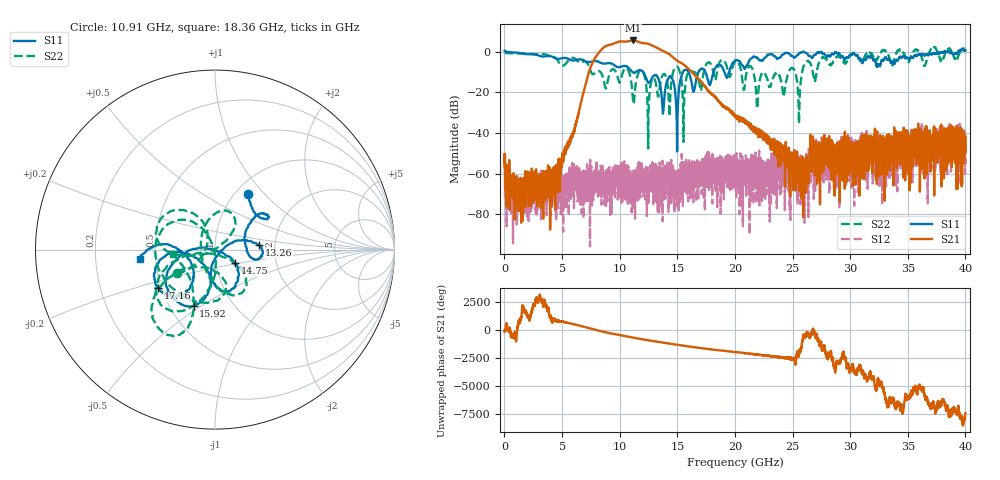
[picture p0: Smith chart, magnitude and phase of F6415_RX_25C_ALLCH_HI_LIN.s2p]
!Keysight Technologies,N5245B,MY52451815,A.15.70.20
!Date: Wednesday, April 17, 2024 14:39:09
!Correction: S33(C  2-Port  )
!S43(C  2-Port  )
!S34(C  2-Port  )
!S44(C  2-Port  )
!S2P File: Measurements: S33, S43, S34, S44:
# Hz S  RI  R 50
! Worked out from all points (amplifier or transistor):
!   4000 points, 10 MHz to 40 GHz, reference 50 ohm
!   highest |S21| = 5.5 dB at 11.15 GHz (marker M1)
!   |S21| within 3 dB of that: 8.712 GHz to 13.02 GHz (4.309 GHz wide, 39.7 % of centre)
!   unconditionally stable (mu >= 1): 139.6 MHz to 25.88 GHz; 25.98 GHz to 32.69 GHz; 35.95 GHz to 36.91 GHz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
!   at 6.67 GHz: K = 4323.53, MAG = -20.5 dB, |S12| = -62.0 dB
!   at 20.01 GHz: K = 8376.42, MAG = -27.7 dB, |S12| = -60.4 dB
!   at 40 GHz: K = 3290.20, MSG = 3.1 dB, |S12| = -55.2 dB
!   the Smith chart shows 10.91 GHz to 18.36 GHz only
!   S11 on the Smith chart (normalised r, x): 10.91 GHz: 1.14, +0.82; 13.26 GHz: 1.64, +0.08; 14.75 GHz: 1.24, -0.19; 15.92 GHz: 0.66, -0.46; 17.16 GHz: 0.48, -0.24; 18.36 GHz: 0.41, -0.05
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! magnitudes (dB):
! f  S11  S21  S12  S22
! 10 MHz  0.5  -54.2  -54.6  -0.7
! 1.41 GHz  -0.7  -65.2  -75.1  -0.9
! 4.24 GHz  -2.7  -67.4  -62.0  -2.6
! 6.68 GHz  -3.9  -24.1  -63.6  -5.3
! 8.22 GHz  -5.2  -0.3  -66.3  -9.6
! 10.91 GHz  -8.8  5.3  -60.4  -12.1
! 11.15 GHz  -10.2  5.5  -67.2  -23.3
! 11.84 GHz  -9.3  4.4  -54.8  -9.2
! 12.45 GHz  -15.2  3.9  -64.7  -37.2
! 13.26 GHz  -12.2  1.8  -64.9  -20.1
! 13.34 GHz  -13.2  1.6  -62.1  -22.0
! 14.75 GHz  -17.3  -3.5  -59.1  -8.3
! 15.54 GHz  -9.5  -6.3  -54.3  -44.4
! 15.92 GHz  -9.5  -8.1  -67.8  -10.5
! 17.16 GHz  -8.3  -15.4  -54.0  -14.9
! 18.36 GHz  -7.5  -22.8  -55.5  -12.6
! 20.01 GHz  -4.4  -31.4  -60.4  -4.9
! 21.94 GHz  -2.9  -39.2  -63.8  -28.0
! 25.75 GHz  -0.4  -56.9  -53.9  -12.8
! 26.67 GHz  -2.9  -44.8  -51.0  -7.7
! 33.34 GHz  -3.4  -51.5  -46.6  -2.1
! 40 GHz  0.5  -49.1  -55.2  1.3
